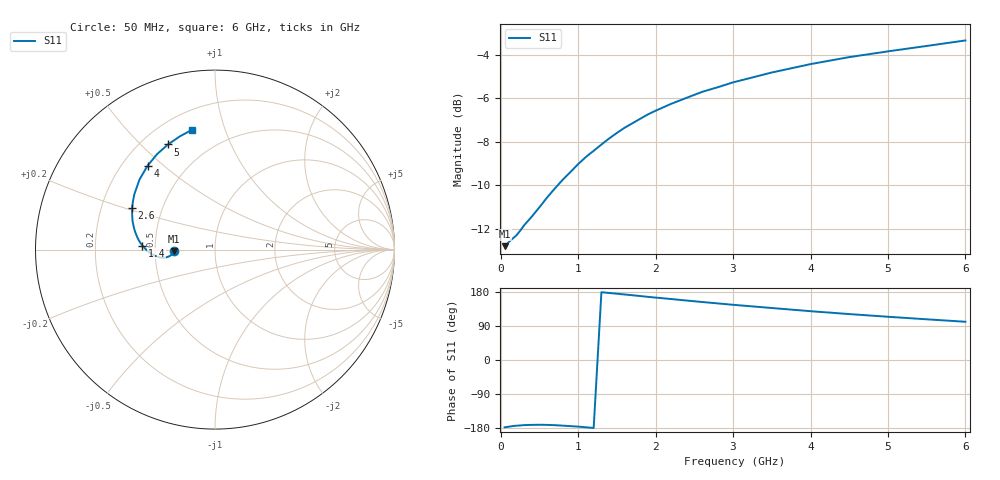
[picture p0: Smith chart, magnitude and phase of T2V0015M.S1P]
! SIEMENS Discrete & RF Semiconductors
! BAS70-04W
! Si Schottky Diode in SOT323
! IF = 15 mA
! S-Parameters:  November  1997
# GHz  S  MA  R  50
!  f  S11
! GHz  MAG  ANG
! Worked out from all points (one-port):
!   34 points, 50 MHz to 6 GHz, reference 50 ohm
!   lowest |S11| = -12.8 dB at 50 MHz (marker M1), VSWR 1.59, Z = 31.4 - j0.635 ohm
!   |S11| at or under -10 dB: start of sweep to 736.9 MHz
!   S11 on the Smith chart (normalised r, x): 50 MHz: 0.63, -0.01; 1.4 GHz: 0.42, +0.02; 2.6 GHz: 0.33, +0.21; 4 GHz: 0.30, +0.44; 5 GHz: 0.30, +0.61; 6 GHz: 0.31, +0.78
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0.05  0.2291 -177.6
0.2  0.2423 -173.4
0.3  0.2556 -171.8
0.4  0.2677 -171.2
0.5  0.2815 -170.9
0.6  0.2965 -171.2
0.7  0.311 -172.0
0.8  0.3254 -173.2
1  0.3537 -175.8
1.1  0.3671 -177.6
1.2  0.3793 -179.4
1.3  0.3921 178.8
1.4  0.4049 176.9
1.6  0.4285 172.9
1.8  0.4491 168.8
1.9  0.4596 166.7
2  0.4688 164.7
2.2  0.4862 160.9
2.4  0.5019 156.9
2.6  0.5179 153.1
2.8  0.5306 149.4
3  0.5446 145.7
3.5  0.5737 137.2
4  0.5998 128.8
4.5  0.6223 121.2
5  0.6415 114.1
5.5  0.6602 107.4
6  0.6796 100.9
